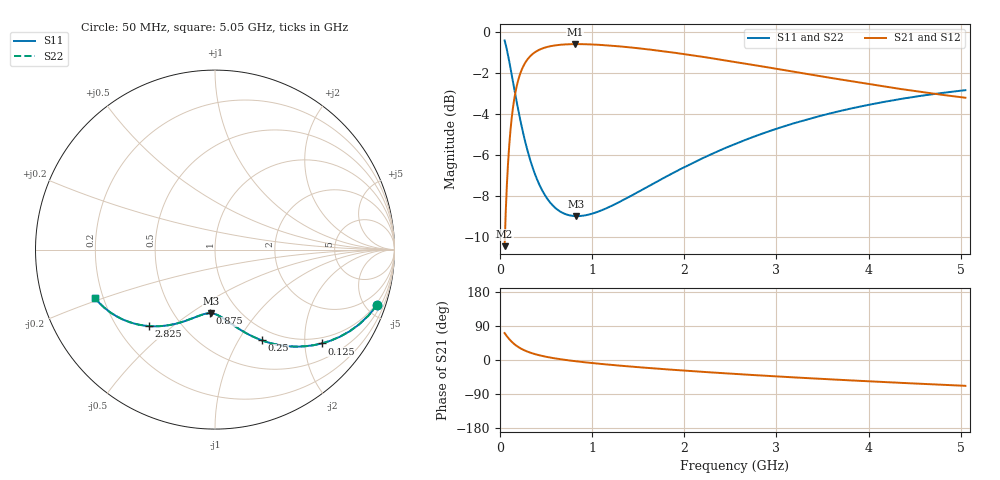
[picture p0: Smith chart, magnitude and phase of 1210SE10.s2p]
! AVX Thin Film Operation		Date: August 2001
! Description: Accu-P® Series, Thin Film, SMD, RF Capacitor
! Part Number: 12101J100FBT
! 50 MHz  -  5.05 GHz
! Serial Measurements
# mhz S db R 50
!	S11		S21		S12		S22
!	dB	Phase	dB	Phase	dB	Phase	dB	Phase
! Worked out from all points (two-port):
!   401 points, 50 MHz to 5.05 GHz, reference 50 ohm
!   highest |S21| = -0.59 dB at 812.5 MHz (marker M1); lowest = -10.5 dB at 50 MHz (marker M2)
!   |S21| within 3 dB of the highest: 144.2 MHz to end of sweep
!   lowest |S11| = -9.0 dB at 825 MHz (marker M3), VSWR 2.10, Z = 37.4 - j30.4 ohm
!   |S11| at or under -10 dB: nowhere
!   |S22| runs from -9.0 to -0.4 dB; largest |S21 - S12| = 0
!   S11 on the Smith chart (normalised r, x): 50 MHz: 0.85, -5.87; 125 MHz: 0.85, -2.39; 250 MHz: 0.84, -1.26; 875 MHz: 0.74, -0.60; 2.825 GHz: 0.33, -0.42; 5.05 GHz: 0.17, -0.19
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50  -0.41 -18.9  -10.45 71.0  -10.45 71.0  -0.41 -18.9
75  -0.87 -27.4  -7.43 62.6  -7.43 62.6  -0.87 -27.4
100  -1.42 -34.9  -5.54 55.1  -5.54 55.1  -1.42 -34.9
125  -2.03 -41.4  -4.28 48.6  -4.28 48.6  -2.03 -41.4
150  -2.65 -47.0  -3.40 43.0  -3.40 43.0  -2.65 -47.0
187.5  -3.56 -54.0  -2.52 36.0  -2.52 36.0  -3.56 -54.0
250  -4.91 -62.8  -1.69 27.2  -1.69 27.2  -4.91 -62.8
337.5  -6.39 -71.3  -1.14 18.7  -1.14 18.7  -6.39 -71.3
450  -7.66 -78.8  -0.82 11.2  -0.82 11.2  -7.66 -78.8
612.5  -8.63 -86.3  -0.64 3.7  -0.64 3.7  -8.63 -86.3
812.5  -8.98 -93.0  -0.59 -3.0  -0.59 -3.0  -8.98 -93.0
825  -8.99 -93.3  -0.59 -3.4  -0.59 -3.4  -8.99 -93.3
875  -8.98 -94.8  -0.59 -4.8  -0.59 -4.8  -8.98 -94.8
887.5  -8.97 -95.1  -0.59 -5.1  -0.59 -5.1  -8.97 -95.1
1262.5  -8.37 -104.1  -0.69 -14.1  -0.69 -14.1  -8.37 -104.1
1725  -7.25 -113.1  -0.91 -23.2  -0.91 -23.2  -7.25 -113.1
2125  -6.32 -120.0  -1.16 -30.1  -1.16 -30.1  -6.32 -120.0
2550  -5.46 -126.7  -1.46 -36.8  -1.46 -36.8  -5.46 -126.7
2825  -4.99 -130.8  -1.66 -40.8  -1.66 -40.8  -4.99 -130.8
3387.5  -4.20 -138.5  -2.09 -48.5  -2.09 -48.5  -4.20 -138.5
4225  -3.36 -148.8  -2.70 -58.9  -2.70 -58.9  -3.36 -148.8
5050  -2.84 -158.1  -3.21 -68.1  -3.21 -68.1  -2.84 -158.1
